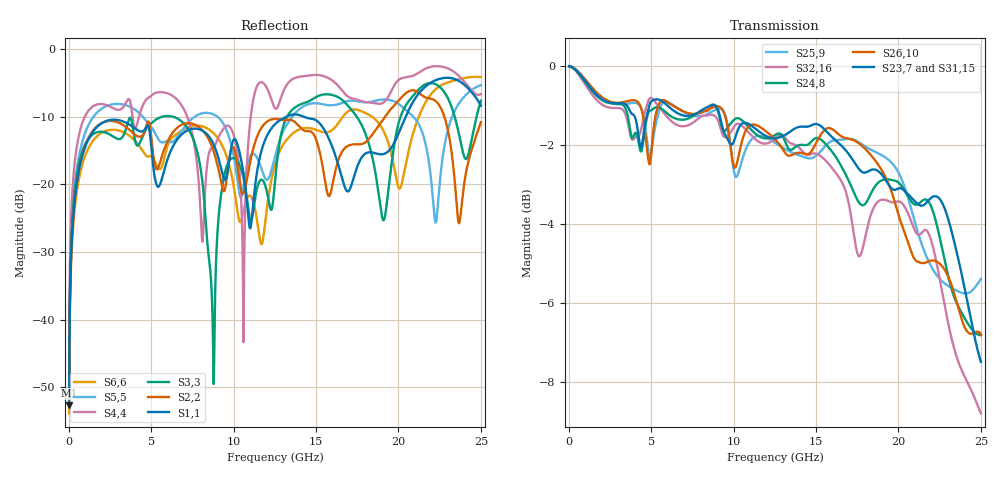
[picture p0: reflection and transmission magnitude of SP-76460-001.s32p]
! Touchstone file from project IMPACT_2P4W_RAvert_100_Ohm_090412
! Exported from HFSS 14.0.0
! Model Description:
! This model is the connector-only, full electrical performance (S-parameter)
! of an Impact Coplanar connector containing 4 wafers, each holding
! 2 differential pairs tuned to 100 ohms and their associated grounds. The
! signal path simulated by the model consists of a right-angle daughter
! card connector mated to a vertical plug header. The model contains
! de-embedded launch structures, but no PCB pads or trace structures are
! included. The electrical model was simulated using Ansoft HFSS in the
! Frequency domain.  This model is designed to highlight
! connector performance and be attached to differential traces in a
! channel model.
! This model can be used as a standalone model for analysis of connector
! performance or with other models to complete a channel.
! Further information regarding this connector series and other related
! Molex connectors can be found at http://www.molex.com/.
! Molex Part Numbers: 76460, 76055
! IMPORTANT NOTE: This model should not be used to evaluate
! electrical signals with greater than 25 GHz of frequency content.
! Please apply appropriate analysis techniques when reviewing the results
! of your simulations.
!               COPYRIGHT 2012, BY MOLEX INCORPORATED
!                 ALL INTERNATIONAL RIGHTS RESERVED
!   THIS FILE CONTAINS MOLEX INCORPORATED CONFIDENTIAL INFORMATION
! >>>>>>>>>>>>>>>>    USER AGREEMENT    <<<<<<<<<<<<<<<<<<<
! The information on this media is the property of MOLEX Incorporated
! and  has been provided to you free of charge. Molex does not
! guarantee that the information is error-free, nor does MOLEX  make
! any representations, warranty or guarantee that the information is
! accurate, correct, reliable or up-to-date. MOLEX expressly
! disclaims all implied warranties regarding this information,
! including but not limited to any implied  warranties of
! merchantability or fitness for a particular purpose. MOLEX does
! not warrant that the media will work correctly in your multi- user
! or network environment.
! MOLEX will in no case be liable for your use, or the results of
! your use, of the software and other information contained on this
! media or  any accompanying written materials.  IT IS YOUR
! RESPONSIBILITY TO VERIFY THE RESULTS OF YOUR USE OF THIS
! INFORMATION IN YOUR OWN PARTICULAR ENGINEERING AND PRODUCT
! ENVIRONMENT, AND YOU ASSUME THE ENTIRE RISK OF DOING SO OR
! FAILING TO DO SO.  In no event will MOLEX be liable for any
! direct, indirect, incidental or consequential damages arising from
! your use of, or your inability to use, software, product simulations
! and other information contained on this media or any accompanying
! written materials.
! This model was solved using HFSS.
! HFSS TDR results can run 5-8 ohms lower than lab results.
! CONNECTION SKETCH
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# GHZ S MA R 50.000000
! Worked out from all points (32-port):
!   2500 points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, 10 MHz to 25 GHz, reference 50 ohm
!   strongest paths, dB at 10 MHz, 6.26 GHz, 12.51 GHz, 18.76 GHz, 25 GHz:
!     S23,7: 0.0, -1.1, -1.8, -2.7, -7.5
!     S31,15: 0.0, -1.3, -2.0, -2.9, -8.0
!     S26,10: 0.0, -1.0, -1.9, -2.5, -6.8
!     S24,8: 0.0, -1.3, -1.7, -3.0, -6.8
!     S32,16: 0.0, -1.4, -1.8, -3.4, -8.8
!     S25,9: 0.0, -1.0, -1.9, -2.2, -5.4
!   lowest |S11| = -52.6 dB at 10 MHz (marker M1), VSWR 1.00, Z = 50 + j0.229 ohm
!   |S11| at or under -10 dB: start of sweep to 13.22 GHz; 14.22 GHz to 20.44 GHz (6.22 GHz wide, 35.9 % of centre)
